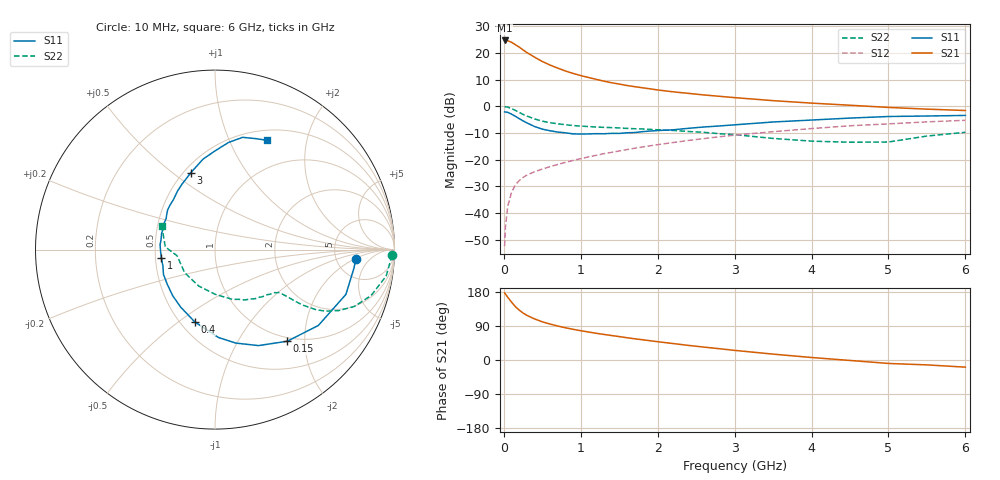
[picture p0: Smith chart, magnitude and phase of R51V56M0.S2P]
! SIEMENS Small Signal Semiconductors
! BFR183
! Si NPN RF Bipolar Junction Transistor in SOT23
! VCE = 1.5 V  IC = 6 mA
! Common Emitter S-Parameters:  May  1996
# GHz  S  MA  R  50
!  f  S11  S21  S12  S22
! GHz  MAG  ANG  MAG  ANG  MAG  ANG  MAG  ANG
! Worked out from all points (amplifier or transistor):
!   36 points, 10 MHz to 6 GHz, reference 50 ohm
!   highest |S21| = 24.7 dB at 10 MHz (marker M1)
!   |S21| within 3 dB of that: start of sweep to 224 MHz
!   unconditionally stable (mu >= 1): 918.2 MHz to 2.647 GHz
!   at 250 MHz: K = 0.48, MSG = 23.9 dB, |S12| = -26.6 dB
!   at 1.4 GHz: K = 1.07, MAG = 11.5 dB, |S12| = -17.3 dB
!   at 6 GHz: K = 0.90, MSG = 1.8 dB, |S12| = -5.2 dB
!   S11 on the Smith chart (normalised r, x): 10 MHz: 7.77, -2.12; 150 MHz: 0.93, -1.65; 400 MHz: 0.59, -0.57; 1 GHz: 0.54, -0.06; 3 GHz: 0.54, +0.58; 6 GHz: 0.62, +1.39
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0.01  0.7862 -3.8  17.12 177.3  0.0024 88.6  0.9863 -1.8
0.02  0.7813 -7.5  17.01 174.1  0.0053 86.5  0.9803 -3.5
0.05  0.7709 -18.9  16.93 165.7  0.0133 80.9  0.9649 -8.8
0.1  0.7143 -36.3  15.83 152.7  0.0244 72.6  0.9065 -16.4
0.15  0.6499 -51.8  14.26 140.8  0.0339 66.3  0.8388 -22.2
0.2  0.5872 -65.6  12.85 131.6  0.0406 62.4  0.7677 -26.3
0.25  0.5335 -77.5  11.38 124.0  0.0466 59.2  0.705 -29.1
0.3  0.4894 -87.9  10.14 117.8  0.0515 57.9  0.657 -30.7
0.4  0.418 -105.7  8.321 108.4  0.0596 56.0  0.5792 -32.3
0.5  0.3733 -120.8  6.909 100.7  0.0668 56.1  0.5262 -32.8
0.6  0.3485 -132.6  5.929 94.9  0.0742 56.7  0.4933 -33.0
0.8  0.319 -154.1  4.593 85.1  0.0889 57.6  0.4514 -33.4
1  0.3024 -171.0  3.763 77.3  0.1047 59.0  0.426 -34.1
1.1  0.3037 -178.8  3.465 73.9  0.1126 59.2  0.4178 -35.1
1.3  0.3058 169.0  2.96 67.5  0.1296 59.1  0.4034 -36.8
1.6  0.3192 153.0  2.453 58.7  0.1547 58.6  0.3858 -40.6
2.2  0.3627 129.5  1.867 43.4  0.2096 55.5  0.3537 -50.6
3  0.4499 107.3  1.454 25.4  0.2882 48.1  0.2942 -70.6
3.5  0.5086 97.5  1.276 15.5  0.3346 42.2  0.2504 -89.0
4.5  0.6018 82.8  1.047 -1.2  0.4319 29.7  0.2124 -142.6
5.5  0.6581 70.0  0.885 -12.9  0.511 17.4  0.2773 176.9
6  0.6747 64.5  0.834 -18.9  0.5469 9.4  0.3261 155.7
